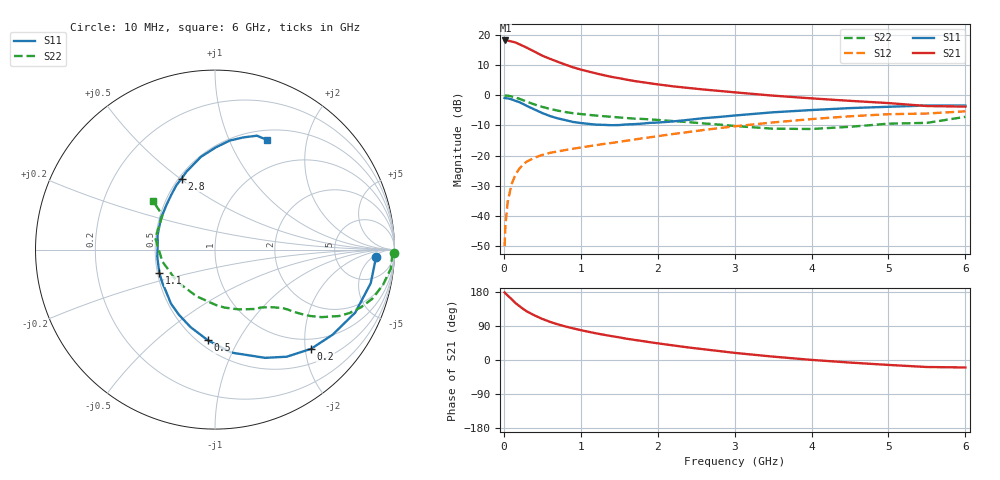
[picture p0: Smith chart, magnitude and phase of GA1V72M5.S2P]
! Infineon Technologies  Discrete & RF Semiconductors
! BF775
! Si NPN RF Bipolar Junction Transistor in SOT23
! VCE = 1.75 V  IC = 2.5 mA
! Common Emitter S-Parameters:  May  1996
# GHz  S  MA  R  50
!  f  S11  S21  S12  S22
! GHz  MAG  ANG  MAG  ANG  MAG  ANG  MAG  ANG
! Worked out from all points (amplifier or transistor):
!   36 points, 10 MHz to 6 GHz, reference 50 ohm
!   highest |S21| = 18.1 dB at 20 MHz (marker M1)
!   |S21| within 3 dB of that: start of sweep to 346 MHz
!   unconditionally stable (mu >= 1): 1.031 GHz to 4.45 GHz; 5.026 GHz to end of sweep
!   at 250 MHz: K = 0.33, MSG = 19.6 dB, |S12| = -22.9 dB
!   at 1.4 GHz: K = 1.14, MAG = 8.6 dB, |S12| = -15.8 dB
!   at 6 GHz: K = 1.02, MAG = 0.0 dB, |S12| = -5.3 dB
!   S11 on the Smith chart (normalised r, x): 10 MHz: 16, -7; 200 MHz: 0.78, -2.12; 500 MHz: 0.56, -0.76; 1.1 GHz: 0.51, -0.15; 2.8 GHz: 0.52, +0.51; 6 GHz: 0.62, +1.39
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0.01  0.8996 -2.5  7.962 178.3  0.0032 88.4  0.9953 -1.2
0.02  0.8938 -4.8  8.047 175.9  0.0069 85.4  0.9875 -2.4
0.05  0.8876 -12.2  8.001 170.1  0.0173 82.1  0.985 -6.2
0.1  0.8565 -24.2  7.738 160.6  0.0336 77.1  0.9566 -11.8
0.15  0.8087 -35.9  7.457 150.5  0.0485 69.8  0.9188 -17.3
0.2  0.7697 -45.9  6.978 142.6  0.0608 65.0  0.8752 -21.5
0.25  0.7182 -56.2  6.52 135.0  0.0717 60.1  0.8294 -25.2
0.3  0.6644 -65.2  6.105 128.1  0.0802 57.1  0.7833 -28.2
0.4  0.5808 -81.0  5.252 117.6  0.0931 51.8  0.7023 -32.4
0.5  0.5073 -94.4  4.508 108.4  0.1034 48.1  0.6422 -35.1
0.6  0.4532 -107.4  4.001 100.7  0.1117 46.3  0.595 -36.9
0.7  0.4147 -119.1  3.577 94.2  0.1178 45.3  0.5572 -38.4
0.9  0.3617 -138.2  2.895 83.5  0.1307 44.5  0.5047 -40.5
1.1  0.3364 -156.9  2.466 74.5  0.1434 44.6  0.4745 -43.0
1.3  0.3239 -173.1  2.144 66.6  0.1566 45.0  0.4501 -45.5
1.6  0.3297 166.0  1.805 56.0  0.1776 45.7  0.4197 -50.1
2.2  0.3691 136.7  1.404 38.5  0.2287 45.3  0.3741 -62.7
2.8  0.4377 115.2  1.179 23.6  0.2862 41.7  0.3274 -80.6
3.5  0.5229 98.6  0.985 8.9  0.3552 34.8  0.2798 -111.6
4.5  0.6131 82.3  0.808 -6.8  0.4488 22.3  0.3009 -167.4
5.5  0.6761 69.8  0.663 -18.5  0.4988 7.2  0.3495 146.8
6  0.6763 64.6  0.649 -19.7  0.5422 3.1  0.4395 141.9
